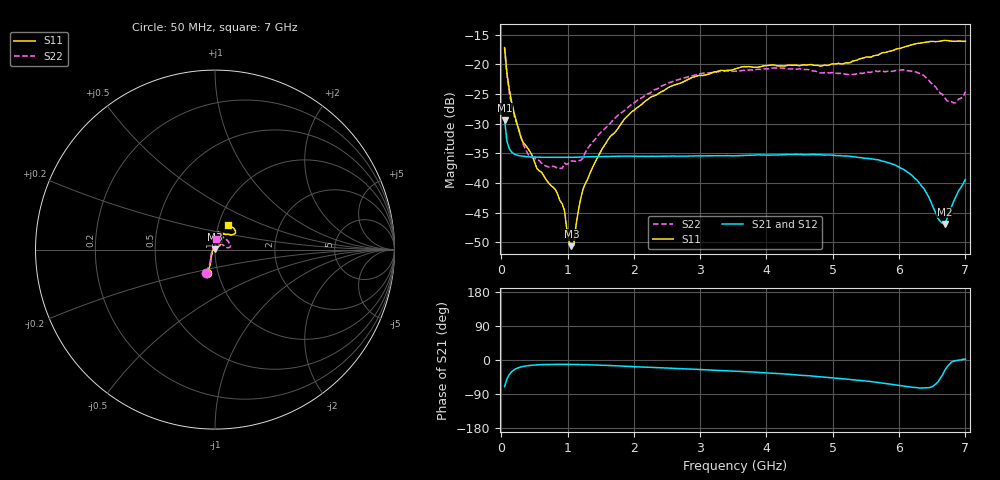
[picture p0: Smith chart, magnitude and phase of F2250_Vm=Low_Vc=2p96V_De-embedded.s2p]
! Integrated Device Technology
! Corporate Headquarters
! 6024 Silver Creek Valley Road
! San Jose, CA 95138  USA
! Phone:  1-408-284-8200
! Toll Free:  1-800-223-1366
! Webpage:  http://www.idt.com/
! Timing and RF Division
! 515 Groton Road, Suite 102
! Westford, MA 01886-6024
! Device:  F2250
! Description: Voltage Variable RF Attenuator
! Frequency:  50.0 -  6000.00 MHz
! Package:  3x3 mm Thin QFN Plastic Package: 16 pin
! Ports:  2 RF, 3 DC
!  Pin  1  = GND
!  Pin  2  = NC
!  Pin  3  = RF1  = Port 1
!  Pin  4  = NC
!  Pin  5  = GND
!  Pin  6  = GND
!  Pin  7  = GND
!  Pin  8  = GND
!  Pin  9  = NC
!  Pin 10  = RF2  = Port 2
!  Pin 11  = NC
!  Pin 12  = GND
!  Pin 13  = GND
!  Pin 14  = VCNTRL
!  Pin 15  = VDD
!  Pin 16  = VMODE
! Vcntrl:  2.960 Volts
! Vmode:  +0.000 Volts
! Vdd:  +3.30  Volts
! Current:  1.176 mA
! Data:  The device was measured on a the F2250 evaluation board which has
!  individual transmission lines to the RF pins.  Data was collected
!  using a calibrated network analyzer.  The evaluation board was
!  de-embedded using a TRL calibration technique.
!  The reference plane is the edge of the package pin.
! Misc:  SN 10
!  Action Tracker AT0258
! Date Measured:  2014-11-26
! Date:  2015-10-15  MJV
! Note:
!  Integrated Device Technology supplies this data as a sample of measured
!  data at the package pin for this product.  Your particular data for this
!  product may vary.
!  Data was taken at 25 degrees C.
!  Integrated Device Technology reserves the right to change this data at anytime.
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# GHz S dB R 50
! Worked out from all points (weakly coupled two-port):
!   201 points, 50 MHz to 7 GHz, reference 50 ohm
!   highest |S21| = -29.41 dB at 50 MHz (marker M1); lowest = -46.9 dB at 6.687 GHz (marker M2)
!   lowest |S11| = -50.6 dB at 1.058 GHz (marker M3), VSWR 1.01, Z = 49.8 + j0.245 ohm
!   |S11| at or under -10 dB: start of sweep to end of sweep
!   |S22| runs from -37.5 to -17.3 dB; largest |S21 - S12| = 5.9e-05
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0.05  -17.18 -108.6  -29.41 -69.8  -29.41 -69.8  -17.28 -111.0
0.08475  -21.45 -107.4  -32.92 -50.3  -32.92 -50.3  -21.75 -110.2
0.15425  -26.23 -116.5  -34.76 -31.1  -34.76 -31.1  -26.81 -122.4
0.29325  -32.22 -128.0  -35.44 -18.5  -35.43 -18.5  -32.11 -137.5
0.3975  -34.11 -142.0  -35.56 -15.0  -35.56 -15.0  -35.03 -160.4
0.91875  -43.51 157.9  -35.68 -11.5  -35.68 -11.5  -37.52 133.4
0.9535  -44.61 170.1  -35.68 -11.5  -35.68 -11.5  -36.64 131.2
1.023  -49.91 143.7  -35.67 -11.6  -35.67 -11.6  -36.62 115.9
1.05775  -50.62 123.4  -35.67 -11.6  -35.67 -11.6  -36.28 110.8
1.0925  -50.49 89.8  -35.66 -11.7  -35.66 -11.7  -36.30 106.3
1.162  -44.66 57.2  -35.64 -11.9  -35.64 -11.9  -36.23 95.4
1.2315  -41.08 44.2  -35.61 -12.1  -35.61 -12.1  -35.80 85.9
1.6485  -32.10 41.9  -35.52 -14.6  -35.52 -14.7  -29.88 64.6
1.96125  -28.05 42.2  -35.46 -17.2  -35.46 -17.2  -26.81 56.8
2.37825  -24.87 47.3  -35.48 -20.3  -35.48 -20.3  -23.99 56.8
3.525  -20.79 72.4  -35.40 -29.5  -35.40 -29.6  -21.18 74.7
4.7065  -20.17 72.3  -35.19 -42.6  -35.19 -42.7  -21.14 72.2
5.85325  -17.81 40.5  -36.63 -63.4  -36.64 -63.5  -21.14 23.1
6.27025  -16.51 40.0  -39.50 -72.8  -39.51 -72.9  -21.37 9.7
6.68725  -16.00 48.7  -46.90 -27.8  -46.86 -27.3  -25.63 28.7
6.861  -16.14 55.1  -42.19 -1.4  -42.15 -1.4  -26.45 57.9
7  -16.13 63.2  -39.38 1.9  -39.33 1.8  -24.63 83.1
